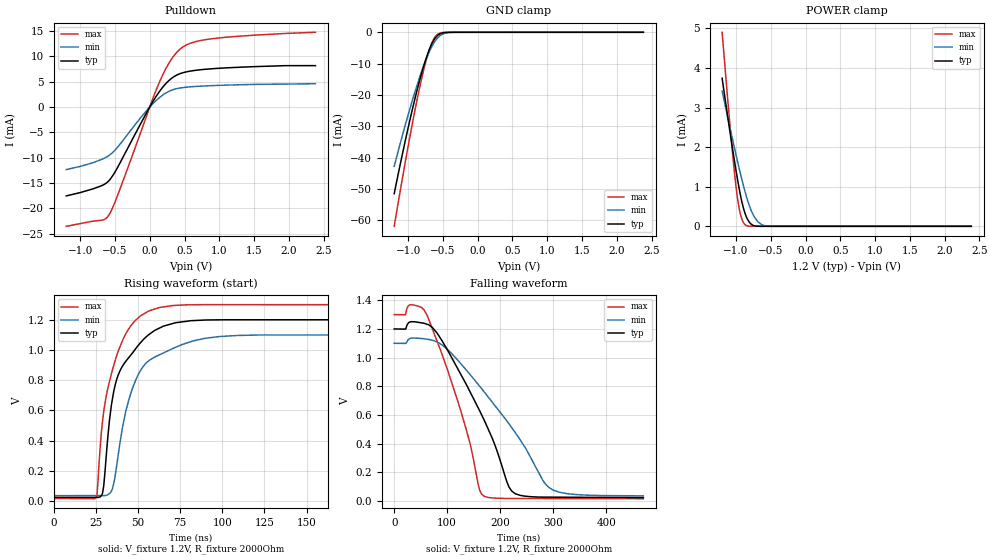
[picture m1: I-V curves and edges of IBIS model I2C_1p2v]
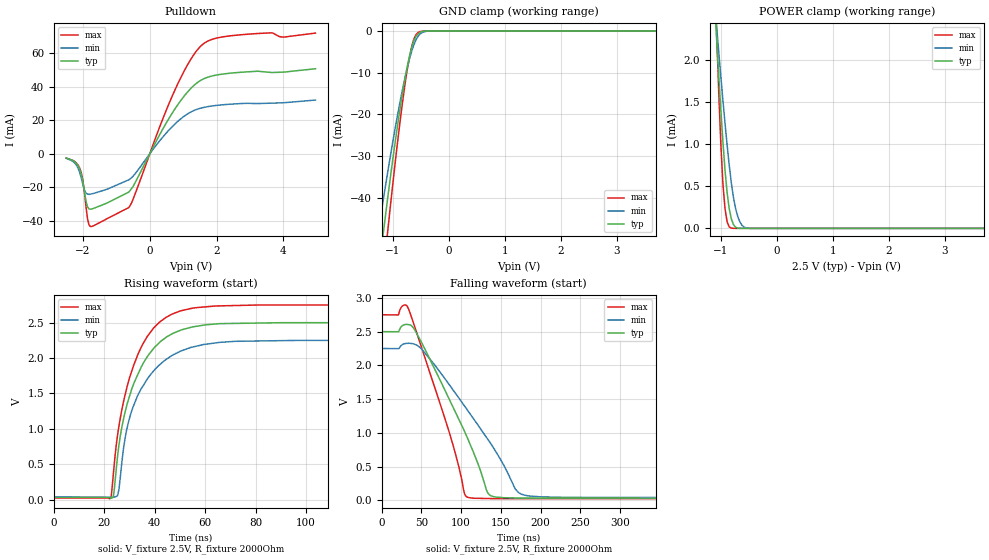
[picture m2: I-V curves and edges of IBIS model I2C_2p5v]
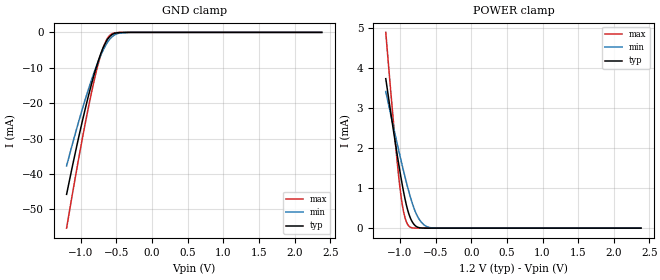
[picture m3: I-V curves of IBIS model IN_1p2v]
|Texas Instruments Incorporated
|Ultra Low Power Stereo Audio Codec With miniDSP, DirectPath Headphone,
|and Class-D Speaker Amplifier
|part#   Digital Voltage Range   Package-type   #pin
|TLV320AIC3268   1.1V to 3.6V   QFN   64
[IBIS Ver]   4.1
[File name]   tlv320aic3268.ibs
[File Rev]   1.0
[Date]   11/21/2013
[Source]   Texas Instruments Incorporated.
   Analog-eLab, HPA
   12500 TI Blvd
   Dallas, TX -75243
   For Support e-mail: elab_ibis@list.ti.com
[Notes]   Revision History:
   1.0: 11/21/2013
- Initial version of the model
- Initial Model generated from simulations.
- Model not matched to measurements
- ccomp values are based on PVT conditions although listed in numerical order.
- Model names with a trailing _1p2v contains the model for 1.2V operaton.
- Model names with a trailing _1p8v contains the model for 1.8V operaton.
- Model names with a trailing _2p5v contains the model for 2.5V operaton.
- Model names with a trailing _3p3v contains the model for 3.3V operaton.
- Warnings regarding pull down/pull up and combined Non-monotonicity of various
  models have been reviewd and considered minor and can be ignored.
[Disclaimer]
 This product is designed as an aid for customers of Texas Instruments.
 No warranties, either expressed or implied, with respect to this third
 party software (if any) or with respect to its fitness for any
 particular purpose is claimed by Texas Instruments or the author. The
 software (if any) is provided solely on an "as is" basis. The entire
 risk as to its quality and performance is with the customer
[Copyright] (C) Copyright 2013 Texas Instruments Incorporated.
   All rights reserved.
|   TLV320AIC3268
[Component]   tlv320aic3268
[Manufacturer] TI
[Package]   | 81 pin  package
| variable   typ   min   max
R_pkg   0.150   0.043   0.221
L_pkg   2.198nH   1.097nH   3.261nH
C_pkg   0.180pF   0.121pF   0.265pF
|-------------------------PIN------------------------------------------------
[Pin]   signal_name  model_name  R_pin  L_pin C_pin
1   GPIO3   INOUT   0.19006   2.76668nH   0.2182pF
2   IOVDD1_33   POWER   0.19998   2.92048nH   0.22549pF
3   MISO_GPO1   OUT   0.19006   2.76668nH   0.2182pF
4   SPI_SELECT   IN_PD   0.17693   2.56318nH   0.20237pF
5   SDA_MOSI   I2C_IO   0.16861   2.43438nH   0.19009pF
6   GPIO5   INOUT   0.1589   2.28438nH   0.16856pF
7   I2C_ADDR_SCLK   IN   0.16617   2.39668nH   0.1782pF
8   SCL_SSZ   I2C_IO   0.15892   2.28468nH   0.18072pF
9   DVDD_18   POWER   0.15135   2.16808nH   0.17011pF
10   IOVDD1_33   POWER   0.1472   2.10478nH   0.16382pF
11   RESETZ   IN   0.14686   2.10038nH   0.16154pF
12   WCLK1   INOUT   0.14973   2.14578nH   0.16441pF
13   GPIO2   INOUT   0.15573   2.23948nH   0.17181pF
14   DOUT1   OUT_HOLD   0.16422   2.37198nH   0.18371pF
15   DIN1   IN   0.17597   2.55508nH   0.19986pF
16   GPIO1   INOUT   0.18998   2.77328nH   0.20201pF
17   BCLK1   INOUT   0.20591   3.02118nH   0.21581pF
18   MCLK   IN   0.19184   2.80268nH   0.20329pF
19   AVDD_18   POWER   0.22137   3.26128nH   0.24656pF
20   IN2L   NC   0.20361   2.98538nH   0.24322pF
21   IN2R   NC   0.18728   2.73188nH   0.21805pF
22   IN3R   NC   0.17455   2.53438nH   0.19914pF
23   IN3L   NC   0.16318   2.35818nH   0.18197pF
24   IN1R_AUX2   NC   0.16065   2.31898nH   0.17764pF
25   IN1L_AUX1   NC   0.1534   2.20668nH   0.16824pF
26   VREF_AUDIO   NC   0.15055   2.16258nH   0.16038pF
27   VREF_SAR   NC   0.14942   2.14518nH   0.16348pF
28   IN4R   NC   0.15128   2.17388nH   0.1692pF
29   IN4L   NC   0.15691   2.26098nH   0.16987pF
30   AVDD1_18   POWER   0.15734   2.26768nH   0.1796pF
31   MICDET   NC   0.16716   2.41988nH   0.19569pF
32   MICBIAS_VDD   NC   0.17556   2.55008nH   0.1947pF
33   MICBIAS_EXT   NC   0.16933   2.45238nH   0.19334pF
34   MICBIAS   NC   0.1476   2.11458nH   0.1658pF
35   RECP   NC   0.16552   2.39348nH   0.18339pF
36   RECVDD_33   NC   0.15324   2.20238nH   0.18332pF
37   RECM   NC   0.13997   1.99608nH   0.15865pF
38   AVDD2_18   POWER   0.12843   1.81668nH   0.14288pF
39   HPR   NC   0.12662   1.78858nH   0.13857pF
40   HVDD_18   POWER   0.12059   1.69438nH   0.1341pF
41   HPL   NC   0.11926   1.67278nH   0.1336pF
42   HPVSS_SENSE   NC   0.12118   1.70128nH   0.13907pF
43   VNEG   NC   0.06276   1.28333nH   0.20934pF
44   CPFCM   NC   0.13055   1.84488nH   0.15526pF
45   CPFCP   NC   0.14318   2.03948nH   0.17067pF
46   CPVDD_18   POWER   0.15898   2.28388nH   0.18816pF
47   LOL   NC   0.17378   2.51318nH   0.2082pF
48   LOR   NC   0.19223   2.79938nH   0.22172pF
49   AVDD4_18   POWER   0.19888   2.90208nH   0.21984pF
50   SPKP   NC   0.04417   1.46589nH   0.22926pF
51   SVDD   POWER   0.04256   1.09698nH   0.26484pF
52   SPKM   NC   0.04407   1.56174nH   0.19503pF
53   SPK_V   NC   0.12258   1.71898nH   0.13283pF
54   VBAT   NC   0.12017   1.68168nH   0.13587pF
55   DVDD_18   POWER   0.11745   1.63958nH   0.12417pF
56   DVSS   GND   0.11639   1.62308nH   0.12233pF
57   DVSS   GND   0.11568   1.61218nH   0.12088pF
58   DOUT2   OUT_HOLD   0.11569   1.61228nH   0.1249pF
59   BCLK2   INOUT   0.11697   1.63208nH   0.13072pF
60   GPIO4   INOUT   0.12223   1.71368nH   0.13702pF
61   DVDD_18   POWER   0.06263   1.20602nH   0.20635pF
62   IOVDD2_33   POWER   0.15368   2.20028nH   0.17922pF
63   DIN2   IN   0.17166   2.47948nH   0.19762pF
64   WCLK2   INOUT   0.19397   2.82638nH   0.21287pF
[Model Selector] I2C_IO
I2C_3p3v   I2C I/O with 3.3V operation.
I2C_2p5v   I2C I/O with 2.5V operation.
I2C_1p8v   I2C I/O with 1.8V operation.
I2C_1p2v   I2C I/O with 1.2V operation.
[Model Selector] IN
IN_3p3v   Input with 3.3V operation.
IN_2p5v   Input with 2.5V operation.
IN_1p8v   Input with 1.8V operation.
IN_1p2v   Input with 1.2V operation.
[Model Selector] IN_PD
IN_PD_3p3v  Input with 3.3V operation.
IN_PD_2p5v  Input with 2.5V operation.
IN_PD_1p8v  Input with 1.8V operation.
IN_PD_1p2v  Input with 1.2V operation.
[Model Selector] INOUT
INOUT_3p3v   I/O with 3.3V operation.
INOUT_2p5v   I/O with 2.5V operation.
INOUT_1p8v   I/O with 1.8V operation.
INOUT_1p2v   I/O with 1.2V operation.
[Model Selector] OUT
OUT_3p3v   Output with 3.3V operation.
OUT_2p5v   Output with 2.5V operation.
OUT_1p8v   Output with 1.8V operation.
OUT_1p2v   Output with 1.2V operation.
[Model Selector] OUT_HOLD
OUT_HOLD_3p3v   Output with 3.3V operation.
OUT_HOLD_2p5v   Output with 2.5V operation.
OUT_HOLD_1p8v   Output with 1.8V operation.
OUT_HOLD_1p2v   Output with 1.2V operation.
| Models and submodels in the file (24): I2C_1p2v (I/O_open_drain), I2C_1p8v (I/O_open_drain), I2C_2p5v (I/O_open_drain), I2C_3p3v (I/O_open_drain), IN_1p2v (Input), IN_1p8v (Input), IN_2p5v (Input), IN_3p3v (Input), IN_PD_1p2v (Input), IN_PD_1p8v (Input), IN_PD_2p5v (Input), IN_PD_3p3v (Input), INOUT_1p2v (I/O), INOUT_1p8v (I/O), INOUT_2p5v (I/O), INOUT_3p3v (I/O), OUT_1p2v (Output), OUT_1p8v (Output), OUT_2p5v (Output), OUT_3p3v (Output), OUT_HOLD_1p2v (Output), OUT_HOLD_1p8v (Output), OUT_HOLD_2p5v (Output), OUT_HOLD_3p3v (Output)
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[Model]   I2C_1p2v
Model_type   I/O_open_drain
Polarity   Non-Inverting
Enable   Active-High
Vinl = 0.12
Vinh = 1.08
Vmeas = 0.6
Vref = 0
Cref = 5pF
Rref = 2000
|   typ   min   max
C_comp   1.274pF   1.219pF   1.333pF
[Voltage Range]   1.2   1.1   1.3
[Temperature Range]   27   125   -40
[Pullup Reference]   1.2   1.1   1.3
[Pulldown Reference]   -0   -0   -0
[Power Clamp Reference]   1.2   1.1   1.3
[GND Clamp Reference]   -0   -0   -0
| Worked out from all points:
|   slope of the pulldown table from 0 to 0.18 V, typ, clamps not added: 47.5 ohm
|   GND clamp passes 1 mA (typ) near -0.58 V on its own axis
|   POWER clamp passes 1 mA (typ) near -0.96 V on its own axis
|   falling waveform, V_fixture 1.2V, R_fixture 2000Ohm: 20-80 % time 88.3ns typ, 123ns min, 62.1ns max; typ from 1.2 V to 0.024 V
|   rising waveform, V_fixture 1.2V, R_fixture 2000Ohm: 20-80 % time 14.7ns typ, 15.2ns min, 13.1ns max; typ from 0.024 V to 1.2 V
[Pulldown]
|   Voltage   I(typ)   I(min)   I(max)
-1.2V     -17.52mA   -12.33mA   -23.52mA
-660mV    -15.3mA    -10.14mA   -22.22mA
-588mV    -14.55mA   -9.571mA   -21.32mA
-534mV    -13.56mA   -8.98mA    -19.87mA
-444mV    -11.44mA   -7.63mA    -16.76mA
-84mV     -2.1mA     -1.335mA   -3.236mA
132mV     2.914mA    1.776mA    4.67mA
294mV     5.441mA    3.206mA    9.049mA
456mV     6.677mA    3.793mA    11.64mA
636mV     7.195mA    4.032mA    12.81mA
924mV     7.575mA    4.234mA    13.51mA
2.382V    8.16mA     4.595mA    14.74mA
[GND Clamp]
|   Voltage   I(typ)   I(min)   I(max)
-1.2V     -51.53mA   -42.82mA   -61.95mA
-1.11V    -41.81mA   -35.22mA   -50.18mA
-966mV    -27.21mA   -23.77mA   -32.33mA
-894mV    -20.51mA   -18.48mA   -24.05mA
-822mV    -14.35mA   -13.57mA   -16.43mA
-750mV    -8.941mA   -9.16mA    -9.735mA
-696mV    -5.556mA   -6.287mA   -5.617mA
-642mV    -2.944mA   -3.902mA   -2.598mA
-588mV    -1.249mA   -2.113mA   -881.8uA
-498mV    -172.7uA   -521.4uA   -72.82uA
-372mV    -4.652uA   -38.41uA   -629.2nA
2.382V    0A         0A         0A
[POWER Clamp]
|   Voltage   I(typ)   I(min)   I(max)
-1.2V     3.742mA    3.419mA    4.901mA
-1.074V   2.231mA    2.387mA    2.298mA
-1.002V   1.428mA    1.82mA     1.03mA
-966mV    1.06mA     1.547mA    562.3uA
-930mV    731.2uA    1.283mA    261.4uA
-894mV    461.7uA    1.032mA    95.6uA
-858mV    267uA      798.5uA    24.83uA
-804mV    94.07uA    498uA      2.256uA
-732mV    11.82uA    224.2uA    69.47nA
-660mV    942.6nA    77.54uA    0A
-570mV    25.2nA     10.87uA    0A
2.382V    0A         0A         0A
[Ramp]
R_load = 2000
|   typ   min   max
dV/dt_r   0.705406/1.46932e-008  0.638454/1.52438e-008  0.769932/1.30398e-008
dV/dt_f   0.705409/8.81291e-008   0.63829/1.23398e-007  0.769933/6.21317e-008
[Falling Waveform]
V_fixture = 1.2V
V_fixture_min = 1.1V
V_fixture_max = 1.3V
R_fixture = 2000Ohm
C_fixture = 0F
|   Time   V(typ)   V(min)   V(max)
0s        1.2V       1.1V       1.3V
32.69ns   1.251V     1.136V     1.369V
62.72ns   1.232V     1.128V     1.29V
120.1ns   920.9mV    981.3mV    694.6mV
161.3ns   629.2mV    800.4mV    74.84mV
169.6ns   565.2mV    761.9mV    34.22mV
216.7ns   96.76mV    537mV      17.74mV
228.5ns   51.31mV    476.9mV    17.7mV
299.2ns   27.33mV    77.85mV    17.43mV
470ns     24.32mV    36.18mV    16.78mV
[Rising Waveform]
V_fixture = 1.2V
V_fixture_min = 1.1V
V_fixture_max = 1.3V
R_fixture = 2000Ohm
C_fixture = 0F
|   Time   V(typ)   V(min)   V(max)
0s        24.32mV    35.9mV     16.78mV
24.99ns   24.02mV    35.98mV    20.42mV
29.9ns    136.2mV    36mV       617.3mV
34.13ns   633.5mV    65.85mV    839.6mV
37.53ns   812.9mV    252.1mV    970.6mV
42.58ns   923.8mV    589mV      1.105V
48.06ns   1.001V     786.7mV    1.193V
62.72ns   1.146V     968.9mV    1.282V
109.1ns   1.201V     1.097V     1.301V
470ns     1.2V       1.1V       1.3V
|   I2C_2p5v
[Model]   I2C_2p5v
Model_type   I/O_open_drain
Polarity   Non-Inverting
Enable   Active-High
Vinl = 0.75
Vinh = 1.75
Vmeas = 1.25
Vref = 0
Cref = 5pF
Rref = 2000
|   typ   min   max
C_comp   1.274pF   1.219pF   1.333pF
[Voltage Range]   2.5   2.25   2.75
[Temperature Range]   27   125   -40
[Pullup Reference]   2.5   2.25   2.75
[Pulldown Reference]   -0   -0   -0
[Power Clamp Reference]   2.5   2.25   2.75
[GND Clamp Reference]   -0   -0   -0
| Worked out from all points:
|   slope of the pulldown table from 0 to 0.375 V, typ, clamps not added: 26.4 ohm
|   GND clamp passes 1 mA (typ) near -0.57 V on its own axis
|   POWER clamp passes 1 mA (typ) near -0.96 V on its own axis
|   falling waveform, V_fixture 2.5V, R_fixture 2000Ohm: 20-80 % time 57.5ns typ, 76.1ns min, 43.6ns max; typ from 2.5 V to 0.031 V
|   rising waveform, V_fixture 2.5V, R_fixture 2000Ohm: 20-80 % time 11.8ns typ, 12.5ns min, 11.3ns max; typ from 0.031 V to 2.5 V
[Pulldown]
|   Voltage   I(typ)   I(min)   I(max)
-2.5V     -2.526mA   -2.66mA    -2.537mA
-2.237V   -4.926mA   -5.666mA   -4.77mA
-2.087V   -9.625mA   -11.74mA   -9.035mA
-2.013V   -15.52mA   -17.53mA   -14.79mA
-1.9V     -28.98mA   -23.51mA   -33.15mA
-1.825V   -32.66mA   -24.09mA   -41.94mA
-1.675V   -32.39mA   -23.49mA   -42.71mA
-625mV    -22.72mA   -15.42mA   -31.93mA
725mV     25.83mA    17.19mA    36.69mA
1.55V     43.97mA    27.3mA     64.52mA
2.525V    48.19mA    29.68mA    70.44mA
4.963V    50.63mA    32mA       71.83mA
[GND Clamp]
|   Voltage   I(typ)   I(min)   I(max)
-2.5V     -395.5mA   -330.9mA   -444.7mA
-1.375V   -71.35mA   -58.36mA   -85.71mA
-1.188V   -50.16mA   -41.75mA   -60.29mA
-1.15V    -46.08mA   -38.56mA   -55.36mA
-1.113V   -42.07mA   -35.43mA   -50.5mA
-1.075V   -38.14mA   -32.35mA   -45.71mA
-887.5mV  -19.93mA   -18.02mA   -23.34mA
-737.5mV  -8.099mA   -8.458mA   -8.701mA
-625mV    -2.309mA   -3.27mA    -1.918mA
-550mV    -742.7uA   -1.242mA   -338.4uA
-287.5mV  -254.6nA   -5.008uA   -31.57nA
4.963V    0A         0A         0A
[POWER Clamp]
|   Voltage   I(typ)   I(min)   I(max)
-2.5V     20.66mA    14.8mA     34.71mA
-1.113V   2.682mA    2.698mA    3.063mA
-1.075V   2.242mA    2.395mA    2.317mA
-1V       1.406mA    1.805mA    1mA
-962.5mV  1.026mA    1.521mA    525.7uA
-925mV    689.7uA    1.247mA    231.4uA
-887.5mV  420.9uA    988.2uA    76.84uA
-812.5mV  113.7uA    540.4uA    3.319uA
-700mV    3.918uA    146.5uA    40.28nA
-625mV    247.3nA    39.26uA    0A
-512.5mV  0A         2.416uA    0A
4.963V    0A         0A         0A
[Ramp]
R_load = 2000
|   typ   min   max
dV/dt_r   1.48138/1.18177e-008   1.32568/1.24678e-008   1.63535/1.12722e-008
dV/dt_f   1.48139/5.7451e-008   1.32569/7.60824e-008   1.63535/4.35846e-008
[Falling Waveform]
V_fixture = 2.5V
V_fixture_min = 2.25V
V_fixture_max = 2.75V
R_fixture = 2000Ohm
C_fixture = 0F
|   Time   V(typ)   V(min)   V(max)
0s        2.5V       2.25V      2.75V
33.44ns   2.604V     2.327V     2.844V
50.29ns   2.335V     2.241V     2.258V
85.86ns   1.476V     1.7V       973.4mV
104.3ns   1.019V     1.396V     94.24mV
107.1ns   945.1mV    1.35V      51.42mV
133.6ns   106.2mV    901.3mV    26.95mV
168ns     35.18mV    167.6mV    25.37mV
176.8ns   33.5mV     86.17mV    25.34mV
470ns     31.02mV    40.52mV    24.42mV
[Rising Waveform]
V_fixture = 2.5V
V_fixture_min = 2.25V
V_fixture_max = 2.75V
R_fixture = 2000Ohm
C_fixture = 0F
|   Time   V(typ)   V(min)   V(max)
0s        31.02mV    40.52mV    24.42mV
22.61ns   24.73mV    36.32mV    22.9mV
23.85ns   103.7mV    36.09mV    457.1mV
25.36ns   639.4mV    67.87mV    931.3mV
26.72ns   976.1mV    445.2mV    1.224V
29.13ns   1.358V     1.027V     1.608V
33.44ns   1.779V     1.484V     2.061V
41.98ns   2.223V     1.906V     2.509V
54.82ns   2.439V     2.154V     2.703V
470ns     2.5V       2.25V      2.75V
|   IN_1p2v
[Model]   IN_1p2v
Model_type   Input
Vinl = 1.08
Vinh = 0.12
|   typ   min   max
C_comp   1.095pF   1.082pF   1.133pF
[Voltage Range]   1.2   1.1   1.3
[Temperature Range]   27   125   -40
[Power Clamp Reference]   1.2   1.1   1.3
[GND Clamp Reference]   -0   -0   -0
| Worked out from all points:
|   GND clamp passes 1 mA (typ) near -0.58 V on its own axis
|   POWER clamp passes 1 mA (typ) near -0.96 V on its own axis
[GND Clamp]
|   Voltage   I(typ)   I(min)   I(max)
-1.2V     -45.78mA   -37.73mA   -55.33mA
-1.11V    -37.06mA   -30.96mA   -44.72mA
-984mV    -25.55mA   -22.02mA   -30.58mA
-894mV    -18.01mA   -16.12mA   -21.24mA
-822mV    -12.53mA   -11.79mA   -14.42mA
-750mV    -7.751mA   -7.917mA   -8.472mA
-696mV    -4.78mA    -5.405mA   -4.842mA
-642mV    -2.508mA   -3.332mA   -2.212mA
-588mV    -1.053mA   -1.79mA    -741uA
-480mV    -90.52uA   -311.7uA   -33.57uA
-300mV    -348.8nA   -5.721uA   -17.65nA
2.382V    0A         0A         0A
[POWER Clamp]
|   Voltage   I(typ)   I(min)   I(max)
-1.2V     3.742mA    3.419mA    4.901mA
-1.074V   2.231mA    2.387mA    2.298mA
-1.002V   1.428mA    1.82mA     1.03mA
-966mV    1.06mA     1.547mA    562.3uA
-930mV    731.2uA    1.283mA    261.4uA
-894mV    461.8uA    1.032mA    95.61uA
-858mV    267uA      798.5uA    24.84uA
-804mV    94.08uA    498uA      2.263uA
-732mV    11.82uA    224.2uA    76.87nA
-660mV    950.1nA    77.55uA    837.8pA
-570mV    32.74nA    10.88uA    0A
2.382V    0A         0A         0A
